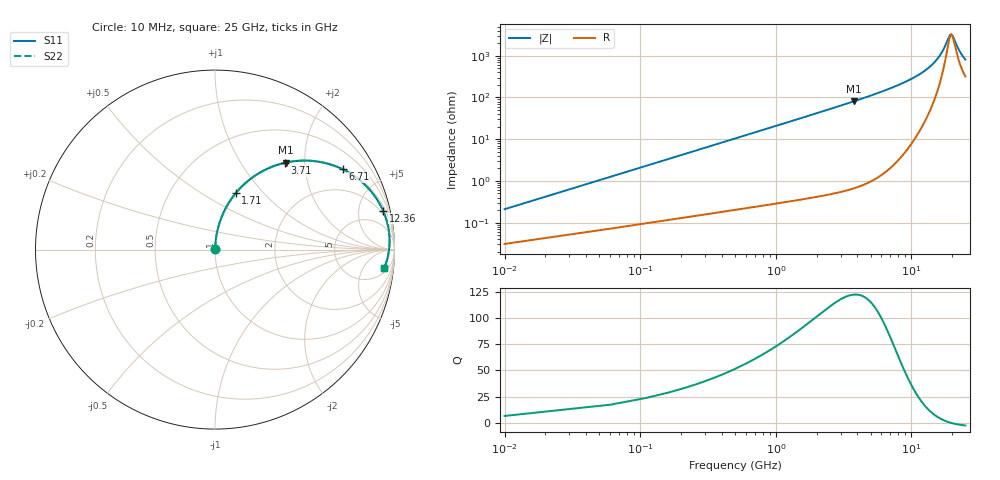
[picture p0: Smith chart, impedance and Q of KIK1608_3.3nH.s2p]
!version-2
!date-04.2020
!Series
# MHz S RI R 50
!Freq ReS11 ImS11 ReS21 ImS21 ReS12 ImS12 ReS22 ImS22
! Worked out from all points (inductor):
!   501 points, 10 MHz to 25 GHz, reference 50 ohm
!   read as one part in series: L = 3.3 nH near 110 MHz
!   highest Q = 122 at 3.76 GHz (marker M1), where L = 3.43 nH
!   self-resonance near 19.74 GHz
!   S11 on the Smith chart (normalised r, x): 10 MHz: 1.00, +0.00; 1.71 GHz: 1.01, +0.71; 3.71 GHz: 1.01, +1.60; 6.71 GHz: 1.04, +3.15; 12.36 GHz: 1.48, +8.45; 25 GHz: 7, -15
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10  0.000313 0.00207  0.9997 -0.00207  0.9997 -0.00207  0.000313 0.00207
160  0.00225 0.0331  0.9978 -0.0331  0.9978 -0.0331  0.00225 0.0331
260  0.00434 0.0536  0.9957 -0.0536  0.9957 -0.0536  0.00434 0.0536
410  0.00897 0.0841  0.991 -0.0841  0.991 -0.0841  0.00897 0.0841
610  0.0179 0.1241  0.9821 -0.1241  0.9821 -0.1241  0.0179 0.1241
910  0.037 0.1816  0.963 -0.1816  0.963 -0.1816  0.037 0.1816
1710  0.1158 0.3147  0.8842 -0.3147  0.8842 -0.3147  0.1158 0.3147
2610  0.2349 0.4195  0.7651 -0.4195  0.7651 -0.4195  0.2349 0.4195
3710  0.3899 0.4836  0.6101 -0.4836  0.6101 -0.4836  0.3899 0.4836
3760  0.3967 0.4851  0.6033 -0.4851  0.6033 -0.4851  0.3967 0.4851
4210  0.4562 0.494  0.5438 -0.494  0.5438 -0.494  0.4562 0.494
6710  0.7107 0.4477  0.2893 -0.4477  0.2893 -0.4477  0.7107 0.4477
8360  0.8135 0.3809  0.1865 -0.3809  0.1865 -0.3809  0.8135 0.3809
12360  0.936 0.2178  0.064 -0.2178  0.064 -0.2178  0.936 0.2178
12510  0.9384 0.2122  0.0616 -0.2122  0.0616 -0.2122  0.9384 0.2122
14860  0.9638 0.132  0.0362 -0.132  0.0362 -0.132  0.9638 0.132
16710  0.9717 0.0769  0.0283 -0.0769  0.0283 -0.0769  0.9717 0.0769
19360  0.9709 0.00884  0.0291 -0.00884  0.0291 -0.00884  0.9709 0.00884
19960  0.9692 -0.00499  0.0308 0.00499  0.0308 0.00499  0.9692 -0.00499
20860  0.9661 -0.0248  0.0339 0.0248  0.0339 0.0248  0.9661 -0.0248
22760  0.9568 -0.0629  0.0432 0.0629  0.0432 0.0629  0.9568 -0.0629
25000  0.9425 -0.1022  0.0575 0.1022  0.0575 0.1022  0.9425 -0.1022
